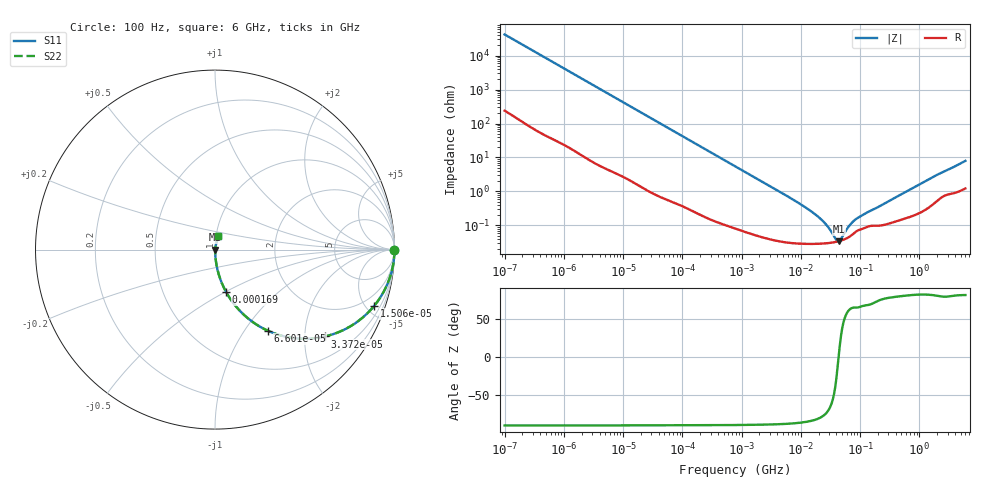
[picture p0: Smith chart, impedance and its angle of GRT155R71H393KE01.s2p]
!Murata Part Number: GRT155R71H393KE01
!These Parameters are Measured in Series Mode Connection
!Data Generated on Jun 19, 2026
!  o--ll--o
!Port1  Port2
!  o------o
!Operation Temp=25[degC], DC Bias Voltage=0[V]
!Freq. Start=100[Hz] Stop=6[GHz] 401[Steps]
# Hz S RI R 50
!Freq.(Hz) S11(Real) S11(Imag) S21(Real) S21(Imag) S12(Real) S12(Imag) S22(Real) S22(Imag)
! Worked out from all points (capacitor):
!   401 points, 100 Hz to 6 GHz, reference 50 ohm
!   read as one part in series: C = 38.1 nF near 109 Hz
!   lowest |Z| = 34.3 mohm at 43.57 MHz (marker M1)
!   series resonance near 43.47 MHz, so ESL is about 350 pH
!   S11 on the Smith chart (normalised r, x): 100 Hz: open; 15.06 kHz: 1.04, -5.63; 33.72 kHz: 1.02, -2.52; 66 kHz: 1.01, -1.29; 169 kHz: 1.00, -0.51; 6 GHz: 1.02, +0.16
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100  1 -0.0024  1.95e-05 0.0024  1.95e-05 0.0024  1 -0.0024
2008  0.9975 -0.0475  0.00253 0.0475  0.00253 0.0475  0.9975 -0.0475
5882  0.9802 -0.1363  0.0198 0.1363  0.0198 0.1363  0.9802 -0.1363
15062  0.8865 -0.3139  0.1135 0.3139  0.1135 0.3139  0.8865 -0.3139
33721  0.6136 -0.4836  0.3864 0.4836  0.3864 0.4836  0.6136 -0.4836
40335  0.527 -0.4959  0.473 0.4959  0.473 0.4959  0.527 -0.4959
66005  0.2962 -0.4527  0.7038 0.4527  0.7038 0.4527  0.2962 -0.4527
103284  0.1485 -0.3513  0.8515 0.3513  0.8515 0.3513  0.1485 -0.3513
169018  0.0625 -0.2374  0.9375 0.2374  0.9375 0.2374  0.0625 -0.2374
774597  0.00391 -0.0556  0.9961 0.0556  0.9961 0.0556  0.00391 -0.0556
6353432  0.000354 -0.00675  0.9996 0.00675  0.9996 0.00675  0.000354 -0.00675
1.555665e7  0.000292 -0.00246  0.9997 0.00246  0.9997 0.00246  0.000292 -0.00246
2.434276e7  0.000296 -0.00124  0.9997 0.00124  0.9997 0.00124  0.000296 -0.00124
3.045065e7  0.000306 -0.000735  0.9997 0.000735  0.9997 0.000735  0.000306 -0.000735
3.80911e7  0.000325 -0.000268  0.9997 0.000268  0.9997 0.000268  0.000325 -0.000268
4.35672e7  0.000342 4.8e-06  0.9997 -4.8e-06  0.9997 -4.8e-06  0.000342 4.8e-06
4.764863e7  0.000358 0.000187  0.9996 -0.000187  0.9996 -0.000187  0.000358 0.000187
6.817316e7  0.000482 0.000938  0.9995 -0.000938  0.9995 -0.000938  0.000482 0.000938
8.527865e7  0.000658 0.00139  0.9993 -0.00139  0.9993 -0.00139  0.000658 0.00139
3.124326e8  0.00117 0.00521  0.9988 -0.00521  0.9988 -0.00521  0.00117 0.00521
1.873145e9  0.00556 0.0284  0.9944 -0.0284  0.9944 -0.0284  0.00556 0.0284
6e9  0.018 0.0763  0.982 -0.0763  0.982 -0.0763  0.018 0.0763
